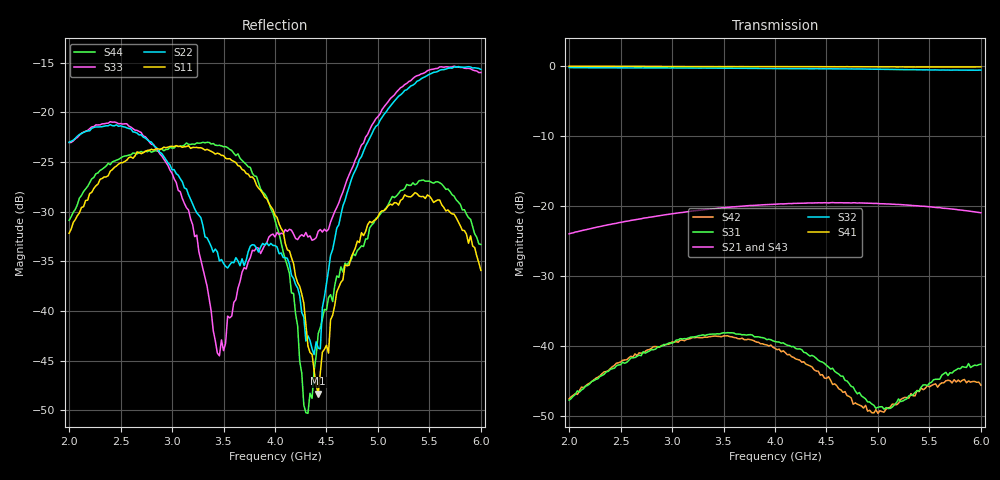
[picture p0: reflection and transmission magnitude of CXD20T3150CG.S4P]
!Agilent Technologies,E5071C,MY46522552,B.13.32
!Date: Tue Dec 24 15:50:18 2024
!Data & Calibration Information:
!Freq	S11:SOLT4(ON)	S12:SOLT4(ON)	S13:SOLT4(ON)	S14:SOLT4(ON)
!	S21:SOLT4(ON)	S22:SOLT4(ON)	S23:SOLT4(ON)	S24:SOLT4(ON)
!	S31:SOLT4(ON)	S32:SOLT4(ON)	S33:SOLT4(ON)	S34:SOLT4(ON)
!	S41:SOLT4(ON)	S42:SOLT4(ON)	S43:SOLT4(ON)	S44:SOLT4(ON)
!PortZ  Port1:50+j0  Port2:50+j0  Port3:50+j0  Port4:50+j0
!Above PortZ is port z conversion or system Z0 setting when saving the data.
!When reading, reference impedance value at option line is always used.
# Hz S dB R 50
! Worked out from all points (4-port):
!   201 points, 2 GHz to 6 GHz, reference 50 ohm
!   strongest paths, dB at 2 GHz, 3 GHz, 4 GHz, 5 GHz, 6 GHz:
!     S41: 0.0, 0.0, -0.1, -0.1, -0.1
!     S32: -0.2, -0.3, -0.3, -0.4, -0.6
!     S21: -23.9, -21.1, -19.7, -19.6, -20.9
!     S43: -23.9, -21.1, -19.7, -19.6, -20.9
!     S31: -47.7, -39.6, -39.3, -48.7, -42.5
!     S42: -47.5, -39.4, -40.3, -49.5, -45.5
!   lowest |S11| = -48.3 dB at 4.42 GHz (marker M1), VSWR 1.01, Z = 50.4 - j0.157 ohm
!   |S11| at or under -10 dB: start of sweep to end of sweep
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2e9  -32.17 84.4  -23.91 56.0  -47.41 86.2  -0.01 -10.3
     -23.93 56.0  -23.00 29.1  -0.19 -56.1  -47.24 87.2
     -47.67 88.9  -0.20 -56.1  -23.02 27.0  -23.90 56.7
     -0.01 -10.3  -47.48 89.0  -23.89 56.7  -30.87 59.2
3.62e9  -25.05 72.0  -20.05 28.6  -37.76 46.1  -0.07 -17.4
        -20.05 28.7  -34.63 -126.7  -0.30 -104.0  -38.94 37.0
        -38.24 45.6  -0.30 -104.0  -38.85 -140.1  -20.05 30.1
        -0.07 -17.5  -38.77 35.8  -20.07 30.2  -24.35 93.7
4.04e9  -31.22 65.1  -19.68 21.0  -39.33 30.9  -0.08 -19.4
        -19.67 21.1  -34.23 -172.4  -0.35 -117.3  -40.38 14.3
        -39.37 27.2  -0.34 -117.3  -32.31 -164.4  -19.66 22.7
        -0.07 -19.3  -40.39 19.7  -19.66 22.6  -32.21 102.7
4.3e9  -41.35 46.3  -19.54 16.3  -41.49 18.3  -0.07 -20.6
       -19.55 16.3  -43.03 -160.9  -0.36 -125.8  -41.40 8.2
       -40.91 16.7  -0.36 -125.6  -32.09 -155.9  -19.54 18.0
       -0.08 -20.6  -42.53 12.3  -19.53 18.0  -50.25 51.3
4.42e9  -48.33 -24.1  -19.51 14.1  -42.38 13.8  -0.07 -21.1
        -19.50 14.0  -43.73 -97.8  -0.35 -129.7  -42.04 6.5
        -41.96 14.2  -0.36 -129.6  -31.98 -135.8  -19.50 16.0
        -0.07 -21.1  -43.52 8.0  -19.51 15.9  -42.27 -41.0
5.1e9  -29.38 -124.7  -19.67 1.5  -47.51 51.4  -0.10 -24.1
       -19.66 1.5  -19.62 -64.2  -0.46 -152.2  -48.33 52.5
       -48.86 53.6  -0.46 -152.2  -18.90 -72.1  -19.66 3.7
       -0.10 -24.2  -48.79 51.0  -19.65 3.7  -29.28 -91.4
6e9  -35.91 -167.9  -20.93 -15.1  -43.52 74.3  -0.09 -28.4
     -20.92 -15.2  -15.66 -96.3  -0.53 177.9  -43.67 50.0
     -42.54 71.2  -0.57 177.9  -15.97 -86.6  -20.91 -12.0
     -0.10 -28.5  -45.52 50.0  -20.90 -12.0  -33.30 -50.6
